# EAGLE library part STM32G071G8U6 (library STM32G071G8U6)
STMICROELECTRONICS - STM32G071G8U6 - MCU, 32BIT, 64MHZ Source: Datasheet
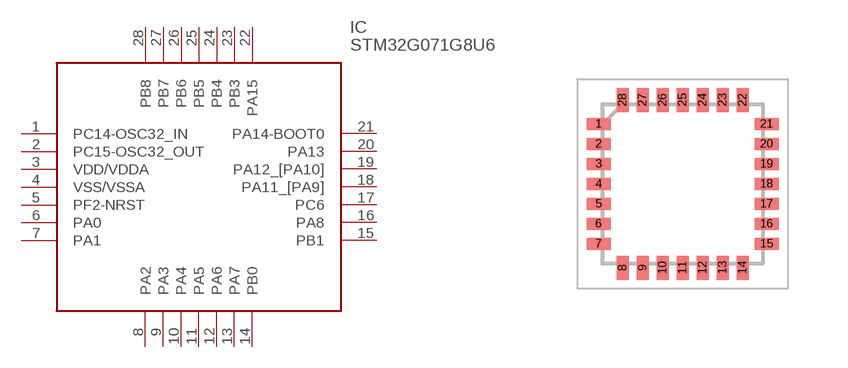
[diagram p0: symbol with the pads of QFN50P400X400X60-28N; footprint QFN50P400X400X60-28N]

Designator prefix IC

## STM32G071G8U6 (Arrow_Part_Number: STM32G071G8U6; Arrow_Price-Stock: https://www.arrow.com/en/products/stm32g071g8u6/stmicroelectronics?utm_currency=USD&region=nac; Description: STMICROELECTRONICS - STM32G071G8U6 - MCU, 32BIT, 64MHZ; Height: 0.6mm; Manufacturer_Name: STMicroelectronics; Manufacturer_Part_Number: STM32G071G8U6; Mouser_Part_Number: 511-STM32G071G8U6; Mouser_Price-Stock: https://www.mouser.co.uk/ProductDetail/STMicroelectronics/STM32G071G8U6?qs=l7cgNqFNU1h6sPpCoQAi5w%3D%3D)  [QFN50P400X400X60-28N]
1  PC14-OSC32_IN
2  PC15-OSC32_OUT
3  VDD/VDDA
4  VSS/VSSA
5  PF2-NRST
6  PA0
7  PA1
8  PA2
9  PA3
10  PA4
11  PA5
12  PA6
13  PA7
14  PB0
15  PB1
16  PA8
17  PC6
18  PA11_[PA9]
19  PA12_[PA10]
20  PA13
21  PA14-BOOT0
22  PA15
23  PB3
24  PB4
25  PB5
26  PB6
27  PB7
28  PB8

## Footprint QFN50P400X400X60-28N (pad centres in mm)
UFQFPN28
smd 0.6 x 0.3: 1 -2.1,1.5; 2 -2.1,1; 3 -2.1,0.5; 4 -2.1,0; 5 -2.1,-0.5; 6 -2.1,-1; 7 -2.1,-1.5; 15 2.1,-1.5; 16 2.1,-1; 17 2.1,-0.5; 18 2.1,0; 19 2.1,0.5; 20 2.1,1; 21 2.1,1.5
smd 0.3 x 0.6: 8 -1.5,-2.1; 9 -1,-2.1; 10 -0.5,-2.1; 11 0,-2.1; 12 0.5,-2.1; 13 1,-2.1; 14 1.5,-2.1; 22 1.5,2.1; 23 1,2.1; 24 0.5,2.1; 25 0,2.1; 26 -0.5,2.1; 27 -1,2.1; 28 -1.5,2.1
